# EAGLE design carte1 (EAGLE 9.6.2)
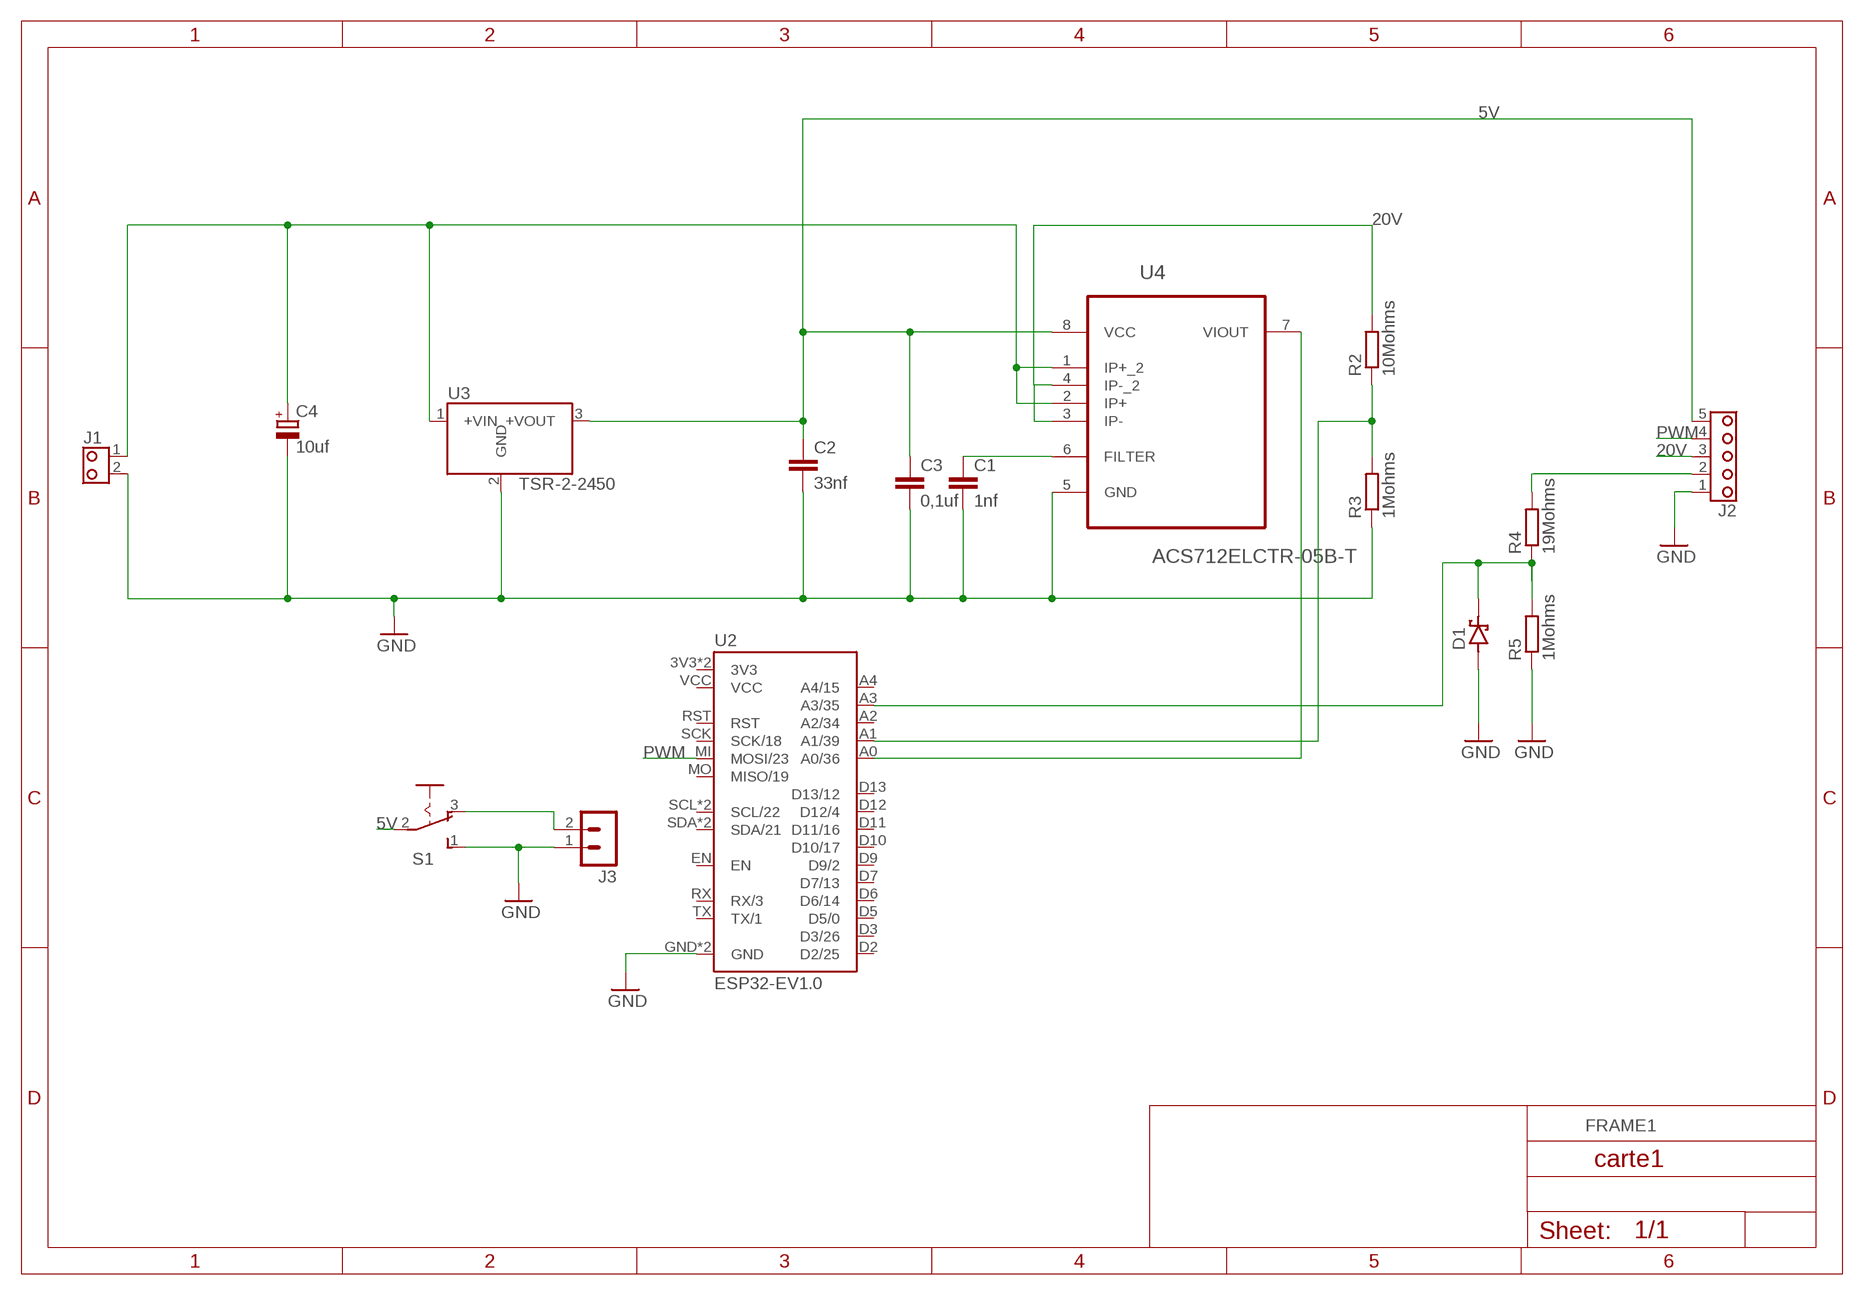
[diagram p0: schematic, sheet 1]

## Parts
C1  1nf  C-C5-3  [C05-3]
C2  33nf  C-C5-3  [C05-3]
C3  0,1uf  C-C5-3  [C05-3]
C4  10uf  C_POL-E5-5  [E5-5]
D1  DIODE_S-DO35  [DO-35-7]
J1  BORNIER_2-D2P  [MSTBA2]
J2  BORNIER_5-D5P  [MSTBA5]
J3  CON2M-PH-KS  [B2B-PH-KS]
R2  10Mohms  R-0207/10  [R0207/10]
R3  1Mohms  R-0207/10  [R0207/10]
R4  19Mohms  R-0207/10  [R0207/10]
R5  1Mohms  R-0207/10  [R0207/10]
S1  1-ON/ON-INTER3  [5636]
U2  ESP32-EV1.0  [ESP32-EV1.0]
U3  TSR-2-2450  [TSR2]
U4  ACS712ELCTR-05B-T  [SOIC127P600X175-8N]

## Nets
5V: C2.1 C3.1 J2.5 S1.2(P) U3.3(+VOUT) U4.8(VCC)
20V: J2.3 R2.2 U4.3(IP-) U4.4(IP-_2)
GND: C1.2 C2.2 C3.2 C4.- D1.A J1.2 J2.1 J3.1 R3.1 R5.1 S1.1(S) U2.GND U2.GNDB(GND) U3.2(GND) U4.5(GND)
N$1: D1.C R4.1 R5.2 U2.A3(A3/35)
N$2: J3.2 S1.3(O)
N$3: C1.1 U4.6(FILTER)
N$4: C4.+ J1.1 U3.1(+VIN) U4.1(IP+_2) U4.2(IP+)
N$5: U2.A0(A0/36) U4.7(VIOUT)
N$7: J2.2 R4.2
N$10: R2.1 R3.2 U2.A1(A1/39)
PWM: J2.4 U2.MI(MOSI/23)
Unconnected: U2.A2(A2/34) U2.A4(A4/15) U2.D2(D2/25) U2.D3(D3/26) U2.D5(D5/0) U2.D6(D6/14) U2.D7(D7/13) U2.D9(D9/2) U2.D10(D10/17) U2.D11(D11/16) U2.D12(D12/4) U2.D13(D13/12) U2.EN U2.MO(MISO/19) U2.RST U2.RX(RX/3) U2.SCK(SCK/18) U2.SCL(SCL/22) U2.SCLB(SCL/22) U2.SDA(SDA/21) U2.SDAB(SDA/21) U2.TX(TX/1)

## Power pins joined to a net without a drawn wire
3V3: U2.3V3 U2.3V3B(3V3)
VCC: U2.VCC

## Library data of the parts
C1-C3 = 0IUT RLCQ:C: Condensateur non Polarisé, Symbole Européen; MAGASIN: (Armoire n°1)
C4 = 0IUT RLCQ:C_POL: Condensateur Polarisé; MAGASIN: (Armoire n°1)
D1 = 0IUT DT:DIODE_S: DIODE Schottky
J1 = 0IUT CONNECTEURS:BORNIER_2: BORNIER, 2 Contacts; MAGASIN: Bornier D2P (Armoire n°4) Bornier D2PF (Armoire n°4)
J2 = 0IUT CONNECTEURS:BORNIER_5: BORNIER, 5 Contacts GEII/IUT ANGERS; MAGASIN: Bornier D5P (Armoire n°4) Bornier D5PF (Armoire n°4)
J3 = 0IUT xPROJETS:CON2M: Connecteur Mâle, 2 Contacts; LIB: CON
R2-R5 = 0IUT RLCQ:R: Résistance Européenne; MAGASIN: (Armoire n°2)
S1 = 0IUT BP INTER:1-ON/ON: 1 Switch ON/ON GEII/IUT ANGERS; MAGASIN: INTER 3 (Armoire n°6)
U2 = 0IUT xPROJETS:ESP32-EV1.0: Module Wifi ESP32-EV1.0 Doc constructeur GEII/IUT ANGERS
U3 = 0IUT xPROJETS:TSR-2-2450: Régulateur de Commutation Tracopower TSR 2 Doc constructeur GEII/IUT ANGERS
U4 = ACS712-05:ACS712ELCTR-05B-T: Linear Current Sensor; MPN: ACS712ELCTR-05B-T; OC_FARNELL: 1329623; OC_NEWARK: 27M3644; PACKAGE: SOIC-8; SUPPLIER: Allegro

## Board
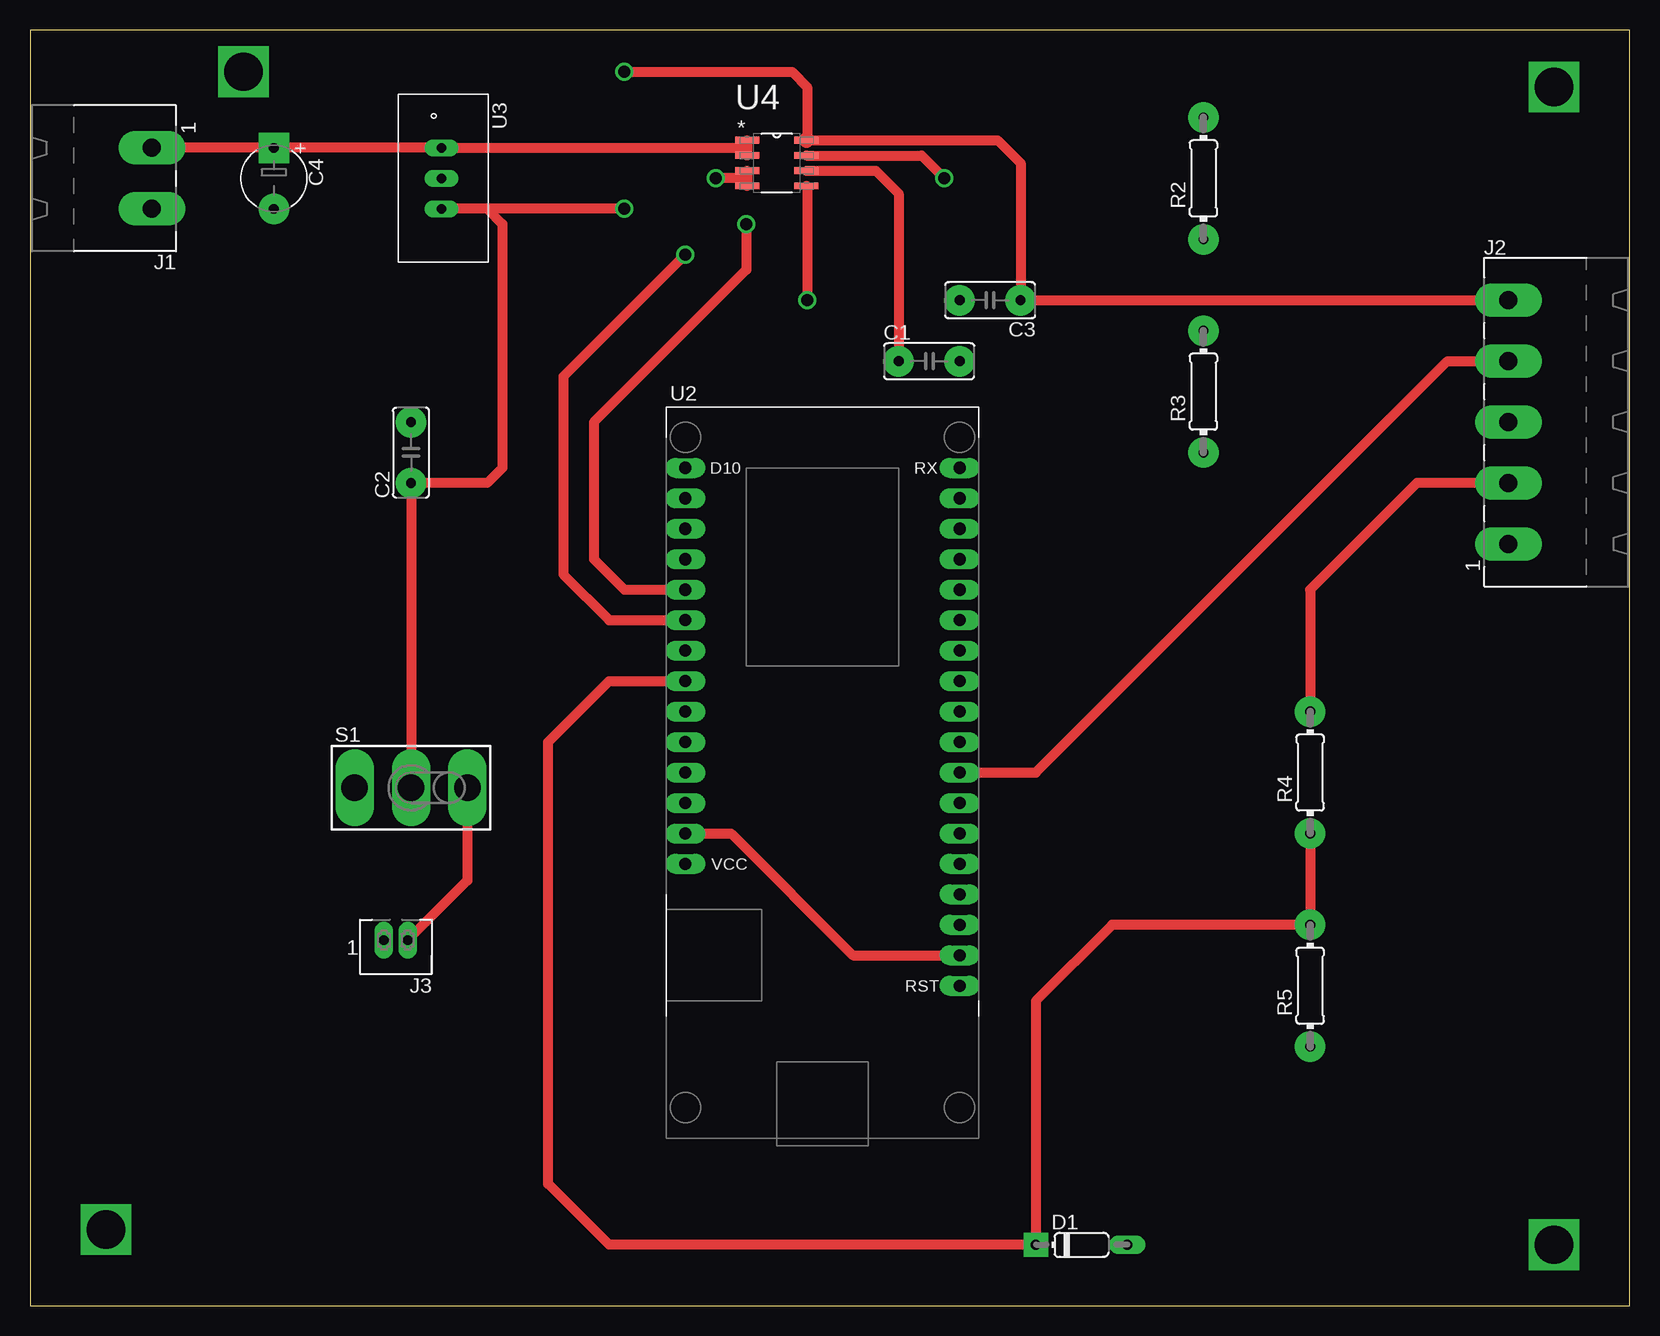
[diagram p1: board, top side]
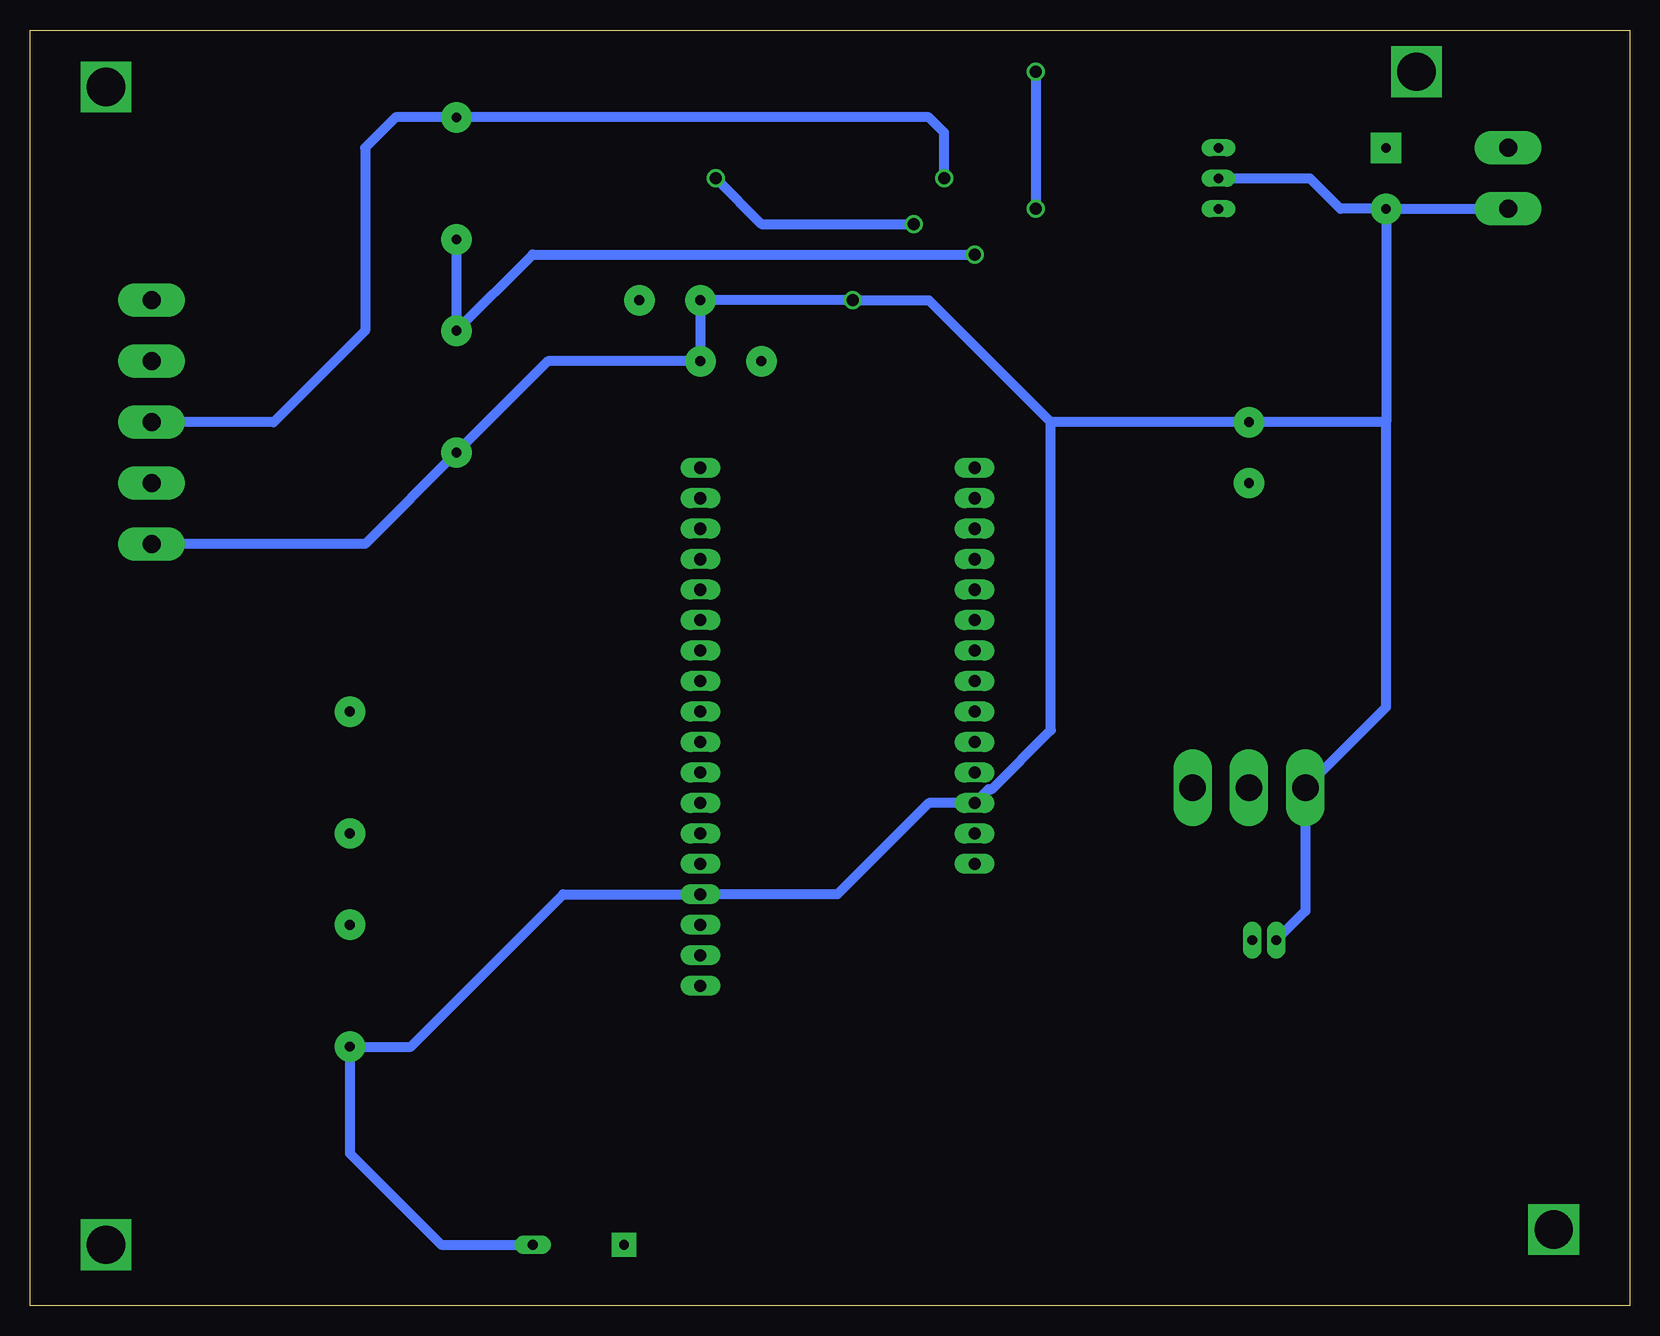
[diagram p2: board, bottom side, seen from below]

Size 133.33 x 106.35 mm. Coordinates in mm from the lower left corner, seen from the top.
Outline: 0,0 133.33,0 133.33,106.35 0,106.35 0,0
Copper layers (1*16): Top 0.035mm / dielectric 1.5mm / Bottom 0.035mm
Design rules "default *": minimum track width 6mil, minimum drill 0.35mm, track to track 6mil, track to pad 6mil, pad to pad 6mil, via to via 6mil, smd to smd 6mil, copper to edge 0mil, drill to drill 6mil, minimum pad ring 10mil, minimum via ring 8mil, stop-mask expansion 4mil, vias tented up to drill 0mil, thermal gap 10mil

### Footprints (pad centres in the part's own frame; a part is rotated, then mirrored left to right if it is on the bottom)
C05-3 = drill 0.813 pad 2.54: 1 -2.54,0; 2 2.54,0
E5-5 = drill 0.813 pad 2.54 square: + -2.54,0 | drill 0.813 pad 2.54: - 2.54,0
DO-35-7 = drill 0.813 pad 1.524 long: A 3.81,0 | drill 0.813 pad 2.032 square: C -3.81,0
MSTBA2 = drill 1.499 pad 2.794 long: 1 -2.54,0; 2 2.54,0
MSTBA5 = drill 1.499 pad 2.794 long: 1 -10.16,0; 2 -5.08,0; 3 0,0; 4 5.08,0; 5 10.16,0
B2B-PH-KS = drill 0.813 pad 1.524 long: 1 1,0; 2 -1,0
R0207/10 = drill 0.813 pad 2.54: 1 -5.08,0; 2 5.08,0
5636 = drill 2.21 pad 2.794 long: 1 -4.699,0; 2 0,0; 3 4.699,0
ESP32-EV1.0 = drill 1.016 pad 1.676 long: 3V3 -11.43,-5.08; 3V3B 11.43,-15.24; A0 -11.43,15.24; A1 -11.43,12.7; A2 -11.43,10.16; A3 -11.43,7.62; A4 -11.43,5.08; D2 11.43,20.32; D3 11.43,17.78; D5 11.43,15.24; D6 11.43,12.7; D7 11.43,10.16; D9 11.43,7.62; D10 -11.43,25.4; D11 -11.43,22.86; D12 -11.43,20.32; D13 -11.43,17.78; EN 11.43,-7.62; GND -11.43,-2.54; GNDB 11.43,-10.16; MI 11.43,0; MO 11.43,-2.54; NC 11.43,-12.7; RST 11.43,-17.78; RX 11.43,25.4; SCK 11.43,-5.08; SCL -11.43,0; SCLB 11.43,2.54; SDA -11.43,2.54; SDAB 11.43,5.08; TX 11.43,22.86; VCC -11.43,-7.62
TSR2 = drill 0.813 pad 1.422 long: 1 -2.54,0; 2 0,0; 3 2.54,0
SOIC127P600X175-8N = smd 1.981 x 0.559: 1 -2.464,1.905; 2 -2.464,0.635; 3 -2.464,-0.635; 4 -2.464,-1.905; 5 2.464,-1.905; 6 2.464,-0.635; 7 2.464,0.635; 8 2.464,1.905

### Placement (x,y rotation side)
C1  74.93,78.74 0 top
C2  31.75,71.12 90 top
C3  80.01,83.82 180 top
C4  20.32,93.98 270 top
D1  87.63,5.08 0 top
J1  10.16,93.98 270 top
J2  123.19,73.66 90 top
J3  30.48,30.48 180 top
R2  97.79,93.98 90 top
R3  97.79,76.2 90 top
R4  106.68,44.45 90 top
R5  106.68,26.67 90 top
S1  31.75,43.18 0 top
U2  66.04,44.45 0 top
U3  34.29,93.98 270 top
U4  62.23,95.25 0 top

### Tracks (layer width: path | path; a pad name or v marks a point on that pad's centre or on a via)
3V3
  Top 0.813: U2.3V3 58.42,39.37 68.58,29.21 U2.3V3B
5V  (via drill 1)
  Top 0.813: v49.53,102.87 63.5,102.87 64.77,101.6 64.77,97.23 | U4.8 80.64,97.16 82.55,95.25 C3.1 J2.5 | S1.2 C2.1 38.1,68.58 39.37,69.85 39.37,90.17 38.1,91.44 | 38.1,91.44 U3.3 | v49.53,91.44 38.1,91.44
  Top 1.27: 64.77,97.23 U4.8
  Bottom 0.813: v49.53,102.87 v49.53,91.44
20V  (via drill 1)
  Top 0.813: U4.3 59.77,93.98 | 59.77,93.98 U4.4 | 59.77,93.98 v57.15,93.98
  Bottom 0.813: J2.3 113.03,73.66 105.41,81.28 105.41,96.52 102.87,99.06 R2.2 58.42,99.06 57.15,97.79 v57.15,93.98
GND  (via drill 1)
  Top 0.813: U4.5 64.77,93.27 v64.77,83.82
  Bottom 0.813: C4.- J1.2 | U3.2 26.67,93.98 24.13,91.44 C4.- | C4.- 20.32,73.66 | 20.32,73.66 C2.2 48.26,73.66 | 48.26,73.66 58.42,83.82 v64.77,83.82 C3.2 C1.2 90.17,78.74 R3.1 105.41,63.5 J2.1 | 48.26,73.66 48.26,47.99 53.19,43.05 53.47,43.05 U2.GND 58.42,41.91 66.04,34.29 U2.GNDB 88.9,34.29 101.6,21.59 R5.1 106.68,12.7 99.06,5.08 D1.A | J3.1 27.05,32.91 S1.1 20.32,49.91 20.32,73.66
N$1
  Top 0.813: R4.1 R5.2 90.17,31.75 83.82,25.4 D1.C 48.26,5.08 43.18,10.16 43.18,46.99 48.26,52.07 U2.A3
N$2
  Top 0.813: S1.3 36.45,35.45 J3.2
N$3
  Top 0.813: U4.6 70.48,94.61 72.39,92.71 C1.1
N$4
  Top 0.813: J1.1 C4.+ U3.1 59.77,96.52 | U4.1 59.77,96.52 | 59.77,96.52 U4.2
N$5  (via drill 1)
  Top 0.813: U4.7 74.3,95.88 v76.2,93.98 | v59.69,90.17 59.69,86.36 46.99,73.66 46.99,62.23 49.53,59.69 U2.A0
  Bottom 0.813: v76.2,93.98 72.39,90.17 v59.69,90.17
N$6  (via drill 3.2)
  other vias: 6.35,6.35
N$7
  Top 0.813: J2.2 115.57,68.58 106.68,59.69 R4.2
N$8  (via drill 3.2)
  other vias: 127,5.08
N$9  (via drill 3.2)
  other vias: 127,101.6
N$10  (via drill 1)
  Top 0.813: U2.A1 48.26,57.15 44.45,60.96 44.45,77.47 v54.61,87.63
  Bottom 0.813: R2.1 R3.2 91.44,87.63 v54.61,87.63
N$11  (via drill 3.2)
  other vias: 17.78,102.87
PWM
  Top 0.813: U2.MI 83.82,44.45 118.11,78.74 J2.4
